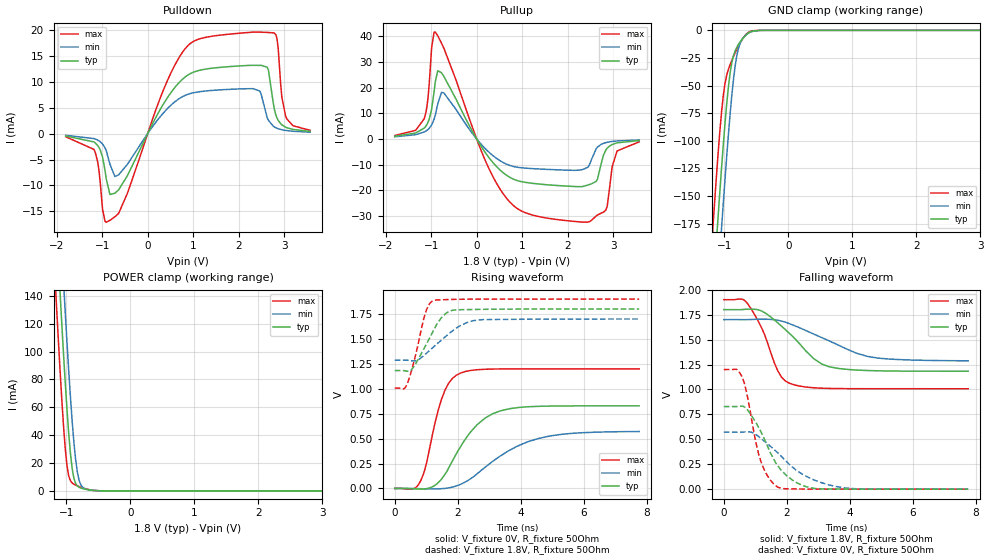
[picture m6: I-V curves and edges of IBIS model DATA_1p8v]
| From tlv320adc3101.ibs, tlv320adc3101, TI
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|   DATA_1p8v
[Model]   DATA_1p8v
Model_type   3-state
Polarity   Non-Inverting
Vmeas = 0.9
Vref = 0
Cref = 5pF
Rref = 1000000
|   typ   min   max
C_comp   1.339pF   1.297pF   1.403pF
[Voltage Range]   1.8   1.7   1.9
[Temperature Range]   27   85   -40
[Pullup Reference]   1.8   1.7   1.9
[Pulldown Reference]   -0   -0   -0
[Power Clamp Reference]   1.8   1.7   1.9
[GND Clamp Reference]   -0   -0   -0
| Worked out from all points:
|   slope of the pulldown table from 0 to 0.27 V, typ, clamps not added: 59 ohm
|   slope of the pullup table from 0 to 0.27 V, typ, clamps not added: 37.3 ohm
|   GND clamp passes 1 mA (typ) near -0.57 V on its own axis
|   POWER clamp passes 1 mA (typ) near -0.68 V on its own axis
|   falling waveform, V_fixture 1.8V, R_fixture 50Ohm: 20-80 % time 1.18ns typ, 1.75ns min, 687ps max; typ from 1.8 V to 1.18 V
|   rising waveform, V_fixture 0V, R_fixture 50Ohm: 20-80 % time 1.06ns typ, 1.65ns min, 567ps max; typ from 0 V to 0.828 V
|   rising waveform, V_fixture 1.8V, R_fixture 50Ohm: 20-80 % time 638ps typ, 947ps min, 402ps max; typ from 1.18 V to 1.8 V
|   falling waveform, V_fixture 0V, R_fixture 50Ohm: 20-80 % time 869ps typ, 1.33ns min, 493ps max; typ from 0.828 V to 0 V
[Pulldown]
|   Voltage   I(typ)   I(min)   I(max)
-1.8V     -446.4uA   -316.7uA   -598.7uA
-1.179V   -1.597mA   -946.4uA   -3.045mA
-936mV    -7.134mA   -2.754mA   -17mA
-828mV    -11.78mA   -5.947mA   -16.77mA
-639mV    -10.88mA   -7.979mA   -15.45mA
792mV     10.74mA    7.283mA    16.07mA
2.331V    13.23mA    8.705mA    19.67mA
2.655V    12.34mA    2.579mA    19.58mA
2.817V    3.684mA    1.156mA    19.18mA
2.952V    1.706mA    765.9uA    6.97mA
3.033V    1.261mA    633.6uA    3.398mA
3.573V    443uA      289.2uA    649.9uA
[GND Clamp]
|   Voltage   I(typ)   I(min)   I(max)
-1.8V     -825.9mA   -883.3mA   -764.9mA
-1.179V   -239.5mA   -297.3mA   -178.5mA
-1.125V   -192mA     -249.1mA   -133mA
-1.098V   -169mA     -225.5mA   -111.7mA
-1.044V   -124.6mA   -179.2mA   -74mA
-990mV    -84.15mA   -134.9mA   -48.1mA
-936mV    -50.69mA   -93.79mA   -35.12mA
-882mV    -28.77mA   -57.92mA   -26.93mA
-828mV    -18.03mA   -30.76mA   -19.85mA
-747mV    -9.84mA    -10.78mA   -10.66mA
-612mV    -2.042mA   -2.193mA   -1.439mA
3.573V    0A         0A         0A
[Pullup]
|   Voltage   I(typ)   I(min)   I(max)
-1.8V     1.069mA    843.6uA    1.356mA
-1.152V   4.248mA    2.71mA     7.898mA
-1.071V   6.407mA    3.659mA    15.68mA
-990mV    11.51mA    5.444mA    35.41mA
-909mV    22.31mA    9.283mA    41.6mA
-720mV    24.33mA    17.9mA     35.29mA
252mV     -6.828mA   -4.846mA   -10.85mA
954mV     -16.5mA    -11.17mA   -27.75mA
2.493V    -17.66mA   -9.482mA   -32.09mA
2.844V    -4.191mA   -1.402mA   -27.56mA
3.087V    -1.512mA   -776.8uA   -4.663mA
3.573V    -627.5uA   -402uA     -1.127mA
[POWER Clamp]
|   Voltage   I(typ)   I(min)   I(max)
-1.8V     799.1mA    851.9mA    743.5mA
-1.179V   212.8mA    267mA      155mA
-1.152V   188.9mA    243mA      131.5mA
-1.098V   142.4mA    195.8mA    86.57mA
-1.044V   98.4mA     150.1mA    46.73mA
-1.017V   77.79mA    128.1mA    30.45mA
-990mV    58.61mA    106.9mA    18.21mA
-909mV    16.07mA    50.13mA    5.734mA
-855mV    5.374mA    22.61mA    4.203mA
-801mV    2.623mA    7.743mA    3.161mA
-450mV    24.48uA    45.72uA    14.68uA
3.573V    0A         0A         0A
[Ramp]
R_load = 50
|   typ   min   max
dV/dt_r   0.497072/1.05808e-009  0.342588/1.65026e-009   0.71977/5.67071e-010
dV/dt_f   0.370361/1.1843e-009   0.24765/1.75289e-009  0.535857/6.87104e-010
[Falling Waveform]
V_fixture = 1.8V
V_fixture_min = 1.7V
V_fixture_max = 1.9V
R_fixture = 50Ohm
C_fixture = 0F
|   Time   V(typ)   V(min)   V(max)
0s        1.8V       1.7V       1.9V
557.9ps   1.8V       1.7V       1.906V
753.7ps   1.805V     1.7V       1.861V
1.201ns   1.786V     1.704V     1.617V
1.717ns   1.667V     1.694V     1.185V
2.096ns   1.558V     1.658V     1.06V
2.86ns    1.307V     1.555V     1.017V
3.356ns   1.226V     1.485V     1.01V
4.905ns   1.187V     1.314V     1.007V
7.76ns    1.183V     1.287V     1.007V
[Rising Waveform]
V_fixture = 0V
V_fixture_min = 0V
V_fixture_max = 0V
R_fixture = 50Ohm
C_fixture = 0F
|   Time   V(typ)   V(min)   V(max)
0s        -6.393uV   -2.606uV   -11.42uV
606.8ps   -4.411mV   -85.13uV   -2.042mV
828ps     -5.61mV    -2.719mV   79.73mV
1.481ns   91.29mV    -2.24mV    892.4mV
1.717ns   208.8mV    6.111mV    1.059V
2.096ns   423.6mV    42.18mV    1.159V
2.86ns    704.5mV    210.3mV    1.196V
3.658ns   800.8mV    385.2mV    1.199V
5.252ns   827.5mV    541.3mV    1.199V
7.76ns    828.4mV    571mV      1.2V
[Rising Waveform]
V_fixture = 1.8V
V_fixture_min = 1.7V
V_fixture_max = 1.9V
R_fixture = 50Ohm
C_fixture = 0F
|   Time   V(typ)   V(min)   V(max)
0s        1.183V     1.286V     1.007V
289.8ps   1.182V     1.287V     1.001V
389ps     1.176V     1.286V     1.045V
606.8ps   1.223V     1.279V     1.269V
921.3ps   1.399V     1.333V     1.706V
1.015ns   1.454V     1.359V     1.798V
1.201ns   1.568V     1.411V     1.883V
1.647ns   1.763V     1.533V     1.895V
2.51ns    1.795V     1.684V     1.899V
7.76ns    1.8V       1.7V       1.9V
[Falling Waveform]
|Gnd
V_fixture = 0V
V_fixture_min = 0V
V_fixture_max = 0V
R_fixture = 50Ohm
C_fixture = 0F
|   Time   V(typ)   V(min)   V(max)
0s        828.4mV    571.6mV    1.2V
400ps     828.4mV    571.4mV    1.201V
557.9ps   832.6mV    571.8mV    1.139V
704.7ps   811.8mV    574.5mV    997.7mV
1.015ns   670mV      548.5mV    473.8mV
1.201ns   560.8mV    503.1mV    256.4mV
1.717ns   234.6mV    363.2mV    19.88mV
2.411ns   49.51mV    166.9mV    1.946mV
3.593ns   1.632mV    24.58mV    174.5uV
7.76ns    1.886uV    79.16uV    -2.995uV
